FUNCTION_BLOCK FB_SignalHandling IMPLEMENTS iSignalHandling
VAR_INPUT
	bInput		AT %I*: BOOL;			// Input signal, e.g. sensor signal, fuse
	bEnable		: BOOL;
END_VAR
VAR_OUTPUT
	bOut		AT %Q* : BOOL;
END_VAR

// =========================================================
;
// =========================================================

METHOD PUBLIC M_SetOutput
VAR_INPUT
END_VAR
// =========================================================
	// Out
	
bOut := bInput AND bEnable;

// =========================================================
END_METHOD

END_FUNCTION_BLOCK
